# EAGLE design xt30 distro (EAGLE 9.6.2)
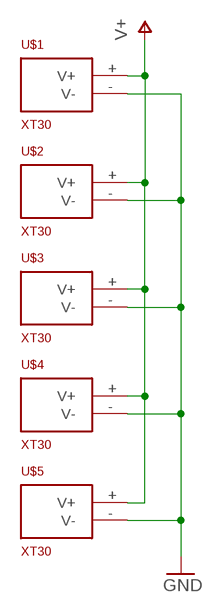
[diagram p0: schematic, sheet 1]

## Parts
U$1  XT30  [XT30]
U$2  XT30  [XT30]
U$3  XT30  [XT30]
U$4  XT30  [XT30]
U$5  XT30  [XT30]

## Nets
GND: U$1.-(V-) U$2.-(V-) U$3.-(V-) U$4.-(V-) U$5.-(V-)
V+: U$1.+(V+) U$2.+(V+) U$3.+(V+) U$4.+(V+) U$5.+(V+)

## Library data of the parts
U$1-U$5 = chris:XT30

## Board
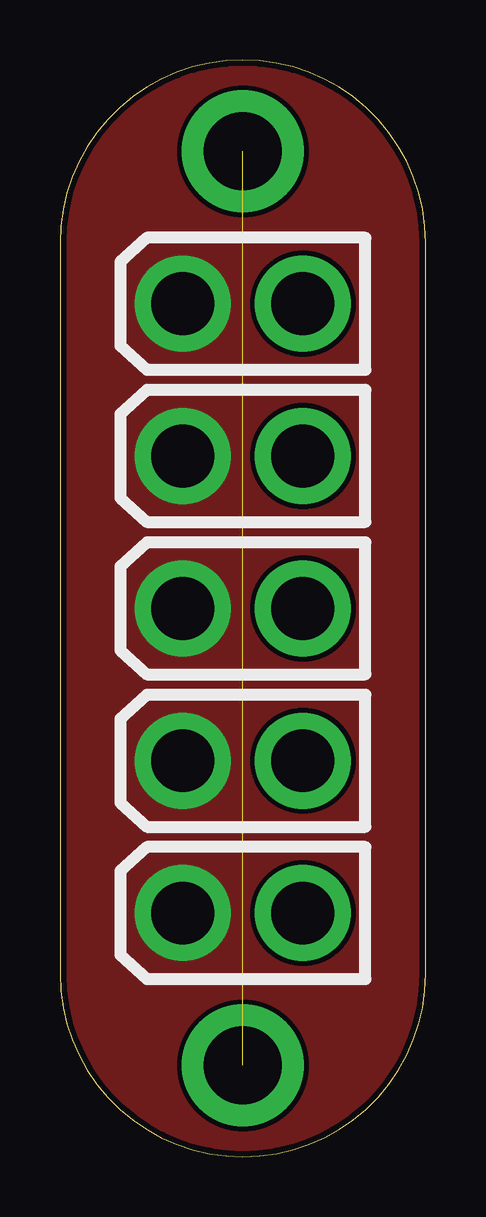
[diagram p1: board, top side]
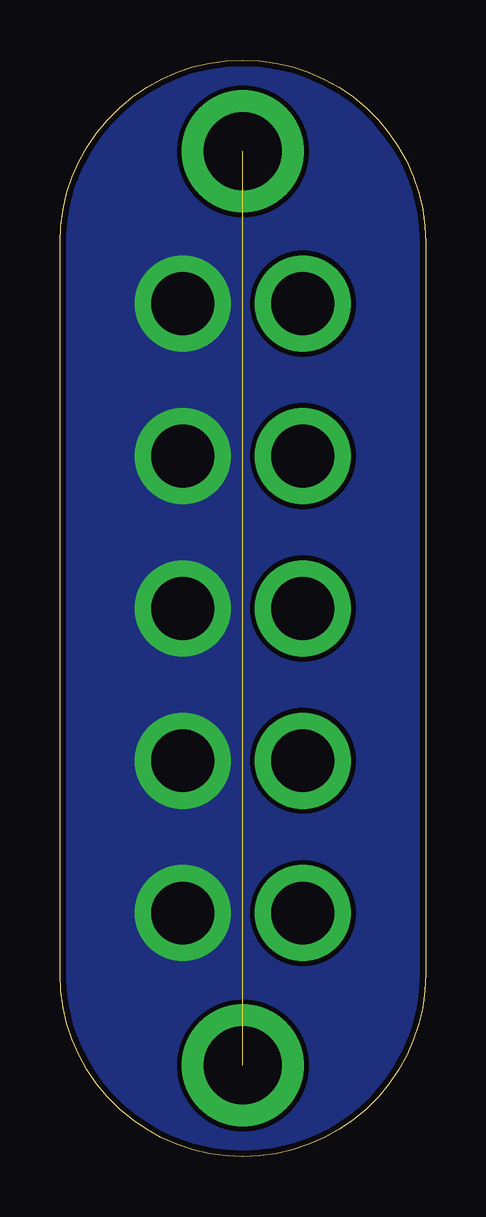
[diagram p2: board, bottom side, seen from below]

Size 15.24 x 45.72 mm. Coordinates in mm from the lower left corner, seen from the top.
Outline: 0,38.1 0,7.62 arc90 7.62,0 arc90 15.24,7.62 15.24,38.1 arc90 7.62,45.72 arc90 0,38.1
Copper layers (1*16): Top 0.035mm / dielectric 1.5mm / Bottom 0.035mm
Design rules "SparkFun": minimum track width 8mil, minimum drill 20mil, track to track 8mil, track to pad 8mil, pad to pad 8mil, via to via 8mil, smd to smd 8mil, copper to edge 10mil, drill to drill 8mil, minimum pad ring 12mil, minimum via ring 10mil, stop-mask expansion 4mil, vias tented up to drill 25mil, thermal gap 10mil

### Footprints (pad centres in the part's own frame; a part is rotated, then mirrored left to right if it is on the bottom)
XT30 = drill 2.62 pad 4: + 2.5,0; - -2.5,0

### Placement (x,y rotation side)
U$1  7.62,10.16 0 top
U$2  7.62,16.51 0 top
U$3  7.62,22.86 0 top
U$4  7.62,29.21 0 top
U$5  7.62,35.56 0 top

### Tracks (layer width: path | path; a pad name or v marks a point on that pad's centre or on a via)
GND
  pour Top (no thermals): -1.27,-1.27 20.32,-1.27 20.32,46.99 -1.27,46.99
N$1  (via drill 3.25 pad 5.08)  (1 unrouted)
  other vias: 7.62,41.91 7.62,3.81
V+
  pour Bottom (no thermals): -2.54,49.53 -2.54,-2.54 22.86,-2.54 22.86,49.53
